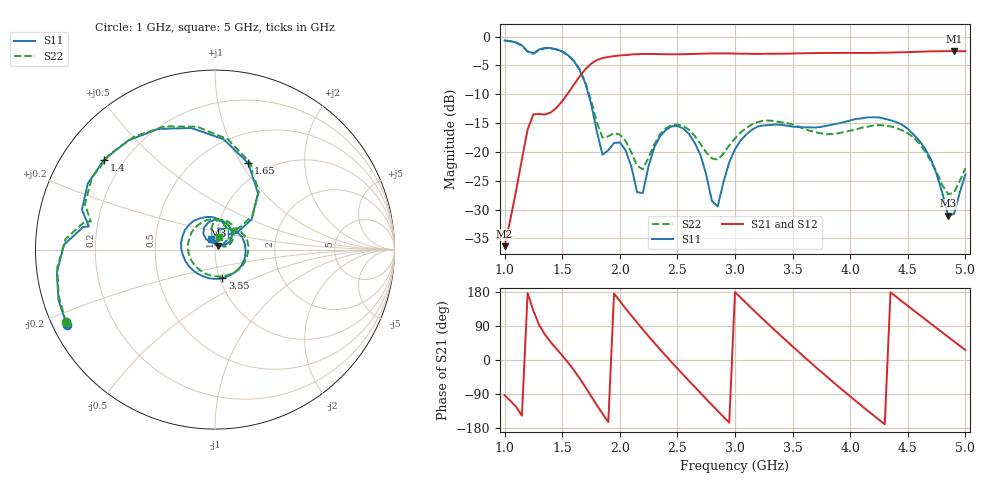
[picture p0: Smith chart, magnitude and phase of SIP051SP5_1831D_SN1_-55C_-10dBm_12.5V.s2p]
# GHz  S  dB  R  50
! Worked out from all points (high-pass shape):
!   81 points, 1 GHz to 5 GHz, reference 50 ohm
!   highest |S21| = -2.51 dB at 4.9 GHz (marker M1); lowest = -36.3 dB at 1 GHz (marker M2)
!   |S21| within 3 dB of the highest: 1.709 GHz to end of sweep
!   lowest |S11| = -31.0 dB at 4.85 GHz (marker M3), VSWR 1.06, Z = 51.8 + j2.2 ohm
!   |S11| at or under -10 dB: 1.728 GHz to end of sweep
!   |S22| runs from -27.3 to -0.7 dB; largest |S21 - S12| = 0.0021
!   S11 on the Smith chart (normalised r, x): 1 GHz: 0.04, -0.24; 1.4 GHz: 0.13, +0.35; 1.65 GHz: 0.82, +1.08; 3.55 GHz: 1.03, -0.34; 5 GHz: 0.95, +0.12
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1  -0.66 -153.0  -36.33 -93.0  -36.23 -93.6  -0.69 -154.1
1.2  -2.55 170.3  -16.09 176.5  -16.08 176.4  -2.60 167.8
1.4  -1.99 140.9  -13.14 47.3  -13.13 47.4  -2.03 138.0
1.65  -5.75 69.0  -6.93 -47.9  -6.93 -47.9  -5.66 67.7
1.7  -8.06 52.7  -5.67 -70.9  -5.67 -70.9  -7.90 52.8
1.85  -20.47 58.7  -3.72 -141.8  -3.72 -141.9  -17.50 56.8
1.95  -18.43 80.5  -3.38 175.6  -3.39 175.5  -16.72 70.0
2.15  -26.97 72.9  -3.04 98.7  -3.05 98.7  -22.39 64.4
2.35  -17.27 116.3  -3.03 27.7  -3.03 27.7  -16.90 94.9
2.5  -15.49 77.3  -3.06 -22.3  -3.06 -22.3  -15.25 66.0
2.7  -20.51 28.4  -2.96 -86.9  -2.95 -86.9  -18.58 37.3
2.85  -29.42 76.3  -2.92 -134.4  -2.92 -134.4  -21.33 54.0
3  -19.53 78.8  -2.94 179.3  -2.93 179.4  -17.62 57.8
3.3  -15.32 -3.6  -2.97 91.5  -2.98 91.5  -14.55 5.4
3.55  -15.67 -75.6  -2.90 22.1  -2.90 22.1  -15.59 -52.7
3.7  -15.76 -114.0  -2.85 -18.4  -2.85 -18.3  -16.60 -94.9
4  -14.54 179.1  -2.82 -96.0  -2.83 -96.1  -16.29 171.6
4.35  -14.51 105.4  -2.76 178.5  -2.78 178.4  -15.57 81.3
4.6  -18.03 54.5  -2.62 119.4  -2.62 119.4  -18.51 31.4
4.85  -31.04 49.3  -2.51 60.9  -2.52 60.9  -27.32 34.5
4.9  -30.77 87.0  -2.51 49.4  -2.51 49.3  -27.07 54.7
5  -23.89 108.9  -2.53 26.2  -2.54 26.2  -22.82 69.8
